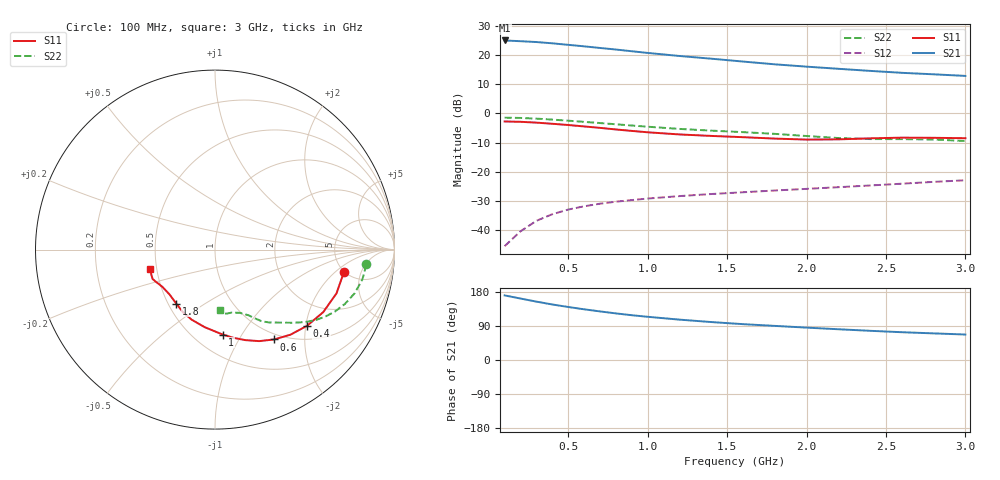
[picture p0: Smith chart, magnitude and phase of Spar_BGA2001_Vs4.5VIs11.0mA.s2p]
! Filename: 4_5G1.001
! Title: BGA2001 X0297-20 HFE=80
! Bias: Vce=4.5V,Ic=11.0mA
! Company: NXP Semiconductors NL
! User: Quality&Reliability T&D
! Measure time: 23 Oct 1998 / 09:22:01
#  MHz  S  MA  R 50
! Freq  S11  S21  S12  S22  :
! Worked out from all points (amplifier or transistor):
!   20 points, 100 MHz to 3 GHz, reference 50 ohm
!   highest |S21| = 25.1 dB at 100 MHz (marker M1)
!   |S21| within 3 dB of that: start of sweep to 778.5 MHz
!   unconditionally stable (mu >= 1): 1.682 GHz to end of sweep
!   at 400 MHz: K = 0.44, MSG = 29.4 dB, |S12| = -34.6 dB
!   at 1.2 GHz: K = 0.80, MSG = 24.1 dB, |S12| = -28.4 dB
!   at 3 GHz: K = 1.25, MAG = 14.9 dB, |S12| = -23.0 dB
!   S11 on the Smith chart (normalised r, x): 100 MHz: 4.93, -2.63; 400 MHz: 1.33, -2.03; 600 MHz: 0.91, -1.43; 1 GHz: 0.68, -0.83; 1.8 GHz: 0.55, -0.38; 3 GHz: 0.46, -0.12
100  0.7291 -9.9  17.99 170.5  0.005239 61.8  0.8471 -5.6
200  0.7195 -19.8  17.47 162.2  0.009434 71.1  0.838 -11.4
300  0.6965 -30.0  16.9 154.0  0.01429 71.3  0.8153 -17.4
400  0.6657 -39.6  16.07 146.6  0.01855 68.9  0.7847 -22.7
500  0.6337 -48.4  15.13 139.9  0.02231 66.2  0.7516 -27.4
600  0.5989 -56.7  14.27 133.8  0.02538 63.9  0.7175 -31.5
700  0.5661 -64.3  13.37 128.2  0.02813 62.1  0.6848 -34.9
800  0.5315 -71.6  12.57 123.0  0.03045 60.4  0.6523 -38.0
900  0.5018 -78.3  11.74 118.2  0.03246 59.5  0.6213 -40.8
1000  0.4751 -84.8  10.99 114.0  0.03446 58.8  0.5924 -43.5
1200  0.4364 -97.4  9.735 106.5  0.038 58.2  0.543 -48.5
1400  0.4114 -108.5  8.747 100.2  0.04126 58.1  0.5074 -53.2
1600  0.3914 -117.3  7.81 94.6  0.04425 58.9  0.478 -56.8
1800  0.3702 -125.7  6.999 90.0  0.04742 60.5  0.4464 -59.5
2000  0.3558 -135.3  6.384 85.5  0.05062 61.2  0.4098 -63.1
2200  0.359 -144.6  5.863 81.2  0.05407 61.5  0.3786 -68.6
2400  0.3736 -151.0  5.399 77.0  0.05785 62.4  0.3632 -75.1
2600  0.3842 -154.7  4.999 73.3  0.06211 63.8  0.3624 -80.0
2800  0.3816 -158.3  4.713 70.2  0.06673 64.0  0.3568 -82.8
3000  0.376 -163.4  4.425 67.2  0.07114 64.5  0.3365 -85.5
